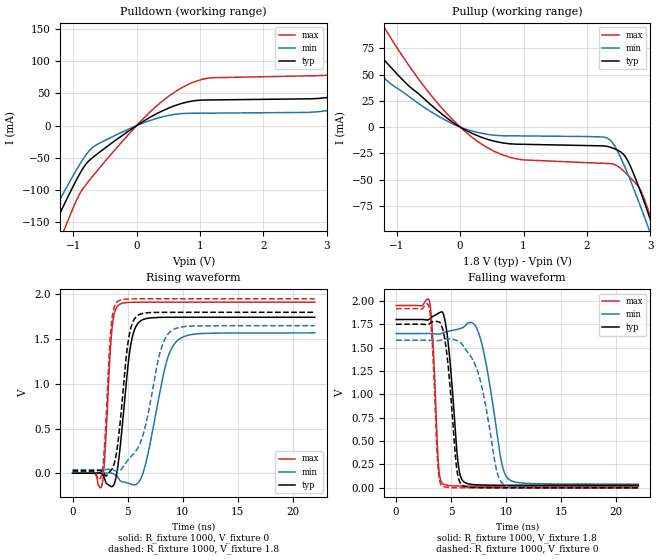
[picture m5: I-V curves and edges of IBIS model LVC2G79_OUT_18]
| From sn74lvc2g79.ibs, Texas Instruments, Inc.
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[Model]   LVC2G79_OUT_18
Model_type  Output
Vref =   0
Rref =   1000
Cref =   30p
Vmeas =   0.9
| variable   typ   min   max
C_comp   9.94pF   6.40pF   16.09pF
| C_pullup   9.15pF   6.40pF   10.36pF
| C_pulldown   10.73pF   6.90pF   16.09pF
[Temperature Range]   40   100   -40
| Ambient temperature   25   85   -40
[Voltage range]   1.8   1.65   1.95
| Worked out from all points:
|   slope of the pulldown table from 0 to 0.27 V, typ, clamps not added: 16.8 ohm
|   slope of the pullup table from 0 to 0.27 V, typ, clamps not added: 33 ohm
|   rising waveform, R_fixture 1000, V_fixture 0: 20-80 % time 863ps typ, 1.55ns min, 502ps max; typ from 0 V to 1.74 V
|   falling waveform, R_fixture 1000, V_fixture 1.8: 20-80 % time 710ps typ, 1.27ns min, 424ps max; typ from 1.8 V to 0.027 V
|   rising waveform, R_fixture 1000, V_fixture 1.8: 20-80 % time 860ps typ, 1.68ns min, 498ps max; typ from 0.027 V to 1.8 V
|   falling waveform, R_fixture 1000, V_fixture 0: 20-80 % time 740ps typ, 1.56ns min, 430ps max; typ from 1.75 V to 0 V
[Pulldown]
| LVC2G79_OUT_18
|   Voltage   I(typ)   I(min)   I(max)
-5.5V     -1.02A     -914.2mA   -1.211A
-1.49V    -194.3mA   -166.1mA   -248.7mA
-1.27V    -148.7mA   -125.7mA   -193.7mA
-1.11V    -116mA     -96.9mA    -154.1mA
-645mV    -45.9mA    -30.54mA   -72.92mA
690mV     33.84mA    18.58mA    57.6mA
3.205V    47.35mA    26.83mA    81.75mA
4.215V    79.09mA    21.52mA    130mA
4.445V    47.14mA    21.65mA    144.9mA
4.62V     44.43mA    21.75mA    152.8mA
5.01V     44.71mA    21.98mA    83.26mA
11V       50.71mA    25.31mA    93.17mA
[Pullup]
| LVC2G79_OUT_18
|   Voltage   I(typ)   I(min)   I(max)
-5.5V     449.7mA    254mA      638.5mA
-2.225V   143.3mA    107.6mA    207.3mA
-1.755V   105.1mA    78.04mA    153.5mA
-1.195V   63.95mA    46.44mA    94.81mA
-375mV    16.75mA    11.48mA    24.15mA
420mV     -11.47mA   -6.842mA   -19.31mA
2.34V     -18.75mA   -11.19mA   -34.79mA
2.61V     -28.71mA   -39.94mA   -43.87mA
2.825V    -58.63mA   -72.76mA   -58mA
2.97V     -83.15mA   -96.31mA   -80.03mA
3.12V     -109.8mA   -121.4mA   -108.9mA
11V       -1.703A    -1.583A    -1.935A
[Ramp]
| LVC2G79_OUT_18
| variable   typ   min   max
dV/dt_r   1.14/9.34E-10   1.02/1.66E-09   1.25/5.44E-10
dV/dt_f   1.11/7.57E-10   1.04/1.40E-09   1.20/4.49E-10
R_load = 1000
[Rising Waveform]
| LVC2G79_OUT_18
R_fixture =   1000
C_fixture =   0
L_fixture =   0
V_fixture =   0
V_fixture_min = 0
V_fixture_max = 0
|   Time   V(typ)   V(min)   V(max)
0s        114pV      8.171nV    2.621nV
2.655ns   -6.993mV   691.8uV    -140.4mV
2.93ns    -66.91mV   2.772mV    193.3mV
3.56ns    -150.3mV   -24.09uV   1.584V
4.235ns   195.3mV    -69.26mV   1.885V
5.24ns    1.401V     -118.9mV   1.911V
6.175ns   1.703V     -67.62mV   1.913V
8.485ns   1.744V     1.224V     1.913V
9.585ns   1.744V     1.49V      1.913V
22ns      1.744V     1.569V     1.913V
[Falling Waveform]
| LVC2G79_OUT_18
R_fixture =   1000
C_fixture =   0
L_fixture =   0
V_fixture =   1.8
V_fixture_min = 1.65
V_fixture_max = 1.95
|   Time   V(typ)   V(min)   V(max)
0s        1.8V       1.65V      1.95V
3.045ns   1.807V     1.65V      1.986V
3.83ns    1.866V     1.644V     278.3mV
4.22ns    1.877V     1.655V     45.06mV
4.78ns    1.49V      1.676V     25.32mV
5.63ns    263.9mV    1.696V     19.59mV
6.125ns   66.09mV    1.718V     18.8mV
7.635ns   30.8mV     1.604V     18.27mV
10.21ns   27.54mV    93.84mV    18.21mV
22ns      27.29mV    39.59mV    18.21mV
[Rising Waveform]
| LVC2G79_OUT_18
R_fixture =   1000
C_fixture =   0
L_fixture =   0
V_fixture =   1.8
V_fixture_min = 1.65
V_fixture_max = 1.95
|   Time   V(typ)   V(min)   V(max)
0s        27.26mV    39.51mV    18.19mV
2.635ns   22.73mV    40.07mV    -16.97mV
2.905ns   -13.79mV   42.1mV     312.1mV
3.495ns   32.85mV    40.81mV    1.63V
4.105ns   327.9mV    20.35mV    1.922V
5.065ns   1.484V     151.5mV    1.948V
5.925ns   1.765V     283.1mV    1.95V
8ns       1.799V     1.375V     1.95V
9.02ns    1.8V       1.597V     1.95V
22ns      1.8V       1.65V      1.95V
[Falling Waveform]
| LVC2G79_OUT_18
R_fixture =   1000
C_fixture =   0
L_fixture =   0
V_fixture =   0
V_fixture_min = 0
V_fixture_max = 0
|   Time   V(typ)   V(min)   V(max)
0s        1.749V     1.578V     1.916V
2.975ns   1.75V      1.578V     1.94V
3.29ns    1.775V     1.576V     1.53V
3.795ns   1.778V     1.574V     231.7mV
4.185ns   1.713V     1.583V     20.55mV
5.49ns    220.7mV    1.576V     1.12mV
5.99ns    29.08mV    1.539V     459.5uV
7.5ns     1.856mV    1.21V      53.78uV
9.71ns    178.3uV    39.88mV    18.57uV
22ns      23.87uV    53.39uV    12.76uV
